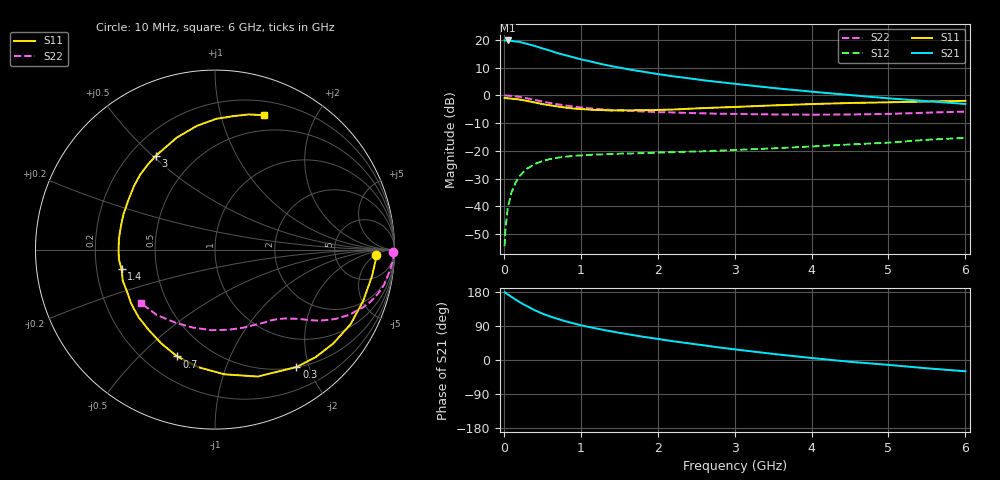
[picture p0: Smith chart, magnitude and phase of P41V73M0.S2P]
! SIEMENS Small Signal Semiconductors
! BFP182
! Si NPN RF Bipolar Junction Transistor in SOT143
! VCE = 1.75 V  IC = 3 mA
! Common Emitter S-Parameters:  March  1996
# GHz  S  MA  R  50
!  f  S11  S21  S12  S22
! GHz  MAG  ANG  MAG  ANG  MAG  ANG  MAG  ANG
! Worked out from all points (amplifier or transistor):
!   36 points, 10 MHz to 6 GHz, reference 50 ohm
!   highest |S21| = 19.8 dB at 50 MHz (marker M1)
!   |S21| within 3 dB of that: start of sweep to 516.8 MHz
!   unconditionally stable (mu >= 1): 1.881 GHz to 5.812 GHz
!   at 250 MHz: K = 0.16, MSG = 23.4 dB, |S12| = -27.8 dB
!   at 1.4 GHz: K = 0.80, MSG = 15.9 dB, |S12| = -21.2 dB
!   at 6 GHz: K = 0.97, MSG = 6.1 dB, |S12| = -15.3 dB
!   S11 on the Smith chart (normalised r, x): 10 MHz: 17, -5; 300 MHz: 0.50, -1.80; 700 MHz: 0.33, -0.65; 1.4 GHz: 0.31, -0.09; 3 GHz: 0.30, +0.51; 6 GHz: 0.34, +1.37
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0.01  0.8952 -1.8  9.785 178.9  0.0019 88.2  0.9942 -0.7
0.02  0.8966 -3.9  9.76 177.9  0.0037 88.1  0.9962 -1.7
0.05  0.887 -9.7  9.802 173.2  0.0092 87.3  0.9908 -4.1
0.1  0.8735 -19.3  9.613 166.5  0.0177 78.5  0.9767 -7.8
0.2  0.8414 -38.5  9.252 153.4  0.0343 68.9  0.9411 -15.1
0.25  0.8203 -47.1  8.865 147.4  0.0409 64.0  0.9148 -18.4
0.3  0.7961 -55.3  8.518 142.3  0.0473 60.1  0.8865 -21.2
0.4  0.7463 -71.4  7.809 131.4  0.0576 52.6  0.8307 -26.0
0.5  0.6968 -85.7  7.049 122.5  0.0651 46.4  0.7747 -29.9
0.6  0.6618 -98.0  6.419 115.0  0.0709 41.8  0.7283 -32.7
0.7  0.6315 -109.5  5.778 108.5  0.0751 37.6  0.691 -34.9
0.8  0.6026 -119.8  5.313 102.3  0.0782 34.1  0.6571 -36.7
0.9  0.5798 -129.8  4.885 97.0  0.0809 31.8  0.6292 -38.2
1.1  0.5557 -147.2  4.178 87.3  0.0843 28.1  0.587 -41.0
1.4  0.5318 -168.2  3.374 75.5  0.0874 24.2  0.5464 -44.6
1.8  0.539 169.0  2.694 61.7  0.0907 22.5  0.5121 -49.6
2.2  0.5554 150.7  2.209 49.5  0.0945 21.3  0.4918 -55.6
3  0.6183 122.1  1.619 28.1  0.1033 21.2  0.4628 -70.1
3.5  0.6595 108.8  1.361 16.1  0.1107 21.0  0.4525 -80.8
4.5  0.7288 89.4  1.014 -4.7  0.13 19.9  0.4514 -105.7
5.5  0.7758 76.1  0.787 -21.9  0.1579 17.0  0.4878 -131.7
6  0.7963 70.1  0.701 -29.7  0.171 13.3  0.5095 -144.4
